ORGANIZATION_BLOCK "I/O Point Fault 2"
TITLE =
VERSION : 0.1


VAR_TEMP
  OB83_EV_CLASS : BYTE ;	//16#38/39, Event class 3, module inserted/removed (8/9)
  OB83_FLT_ID : BYTE ;	//16#XX, Fault identifcation code
  OB83_PRIORITY : BYTE ;	//26/28 (Priority of 1 is lowest)
  OB83_OB_NUMBR : BYTE ;	//83 (Organization block 83, OB83)
  OB83_RESERVED_1 : BYTE ;	//Reserved for system
  OB83_MDL_ID : BYTE ;	//Input module (01010100), Output module (01010101)
  OB83_MDL_ADDR : WORD ;	//Base address of module with point fault
  OB83_RACK_NUM : WORD ;	//Number of rack that has module with point fault
  OB83_MDL_TYPE : WORD ;	//Module type with point fault
  OB83_DATE_TIME : DATE_AND_TIME ;	//Date and time OB83 started
END_VAR
BEGIN
END_ORGANIZATION_BLOCK

